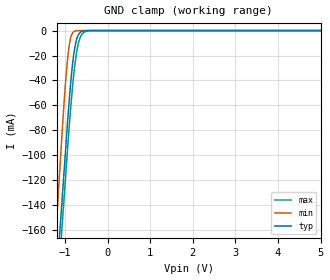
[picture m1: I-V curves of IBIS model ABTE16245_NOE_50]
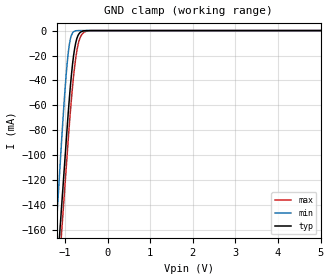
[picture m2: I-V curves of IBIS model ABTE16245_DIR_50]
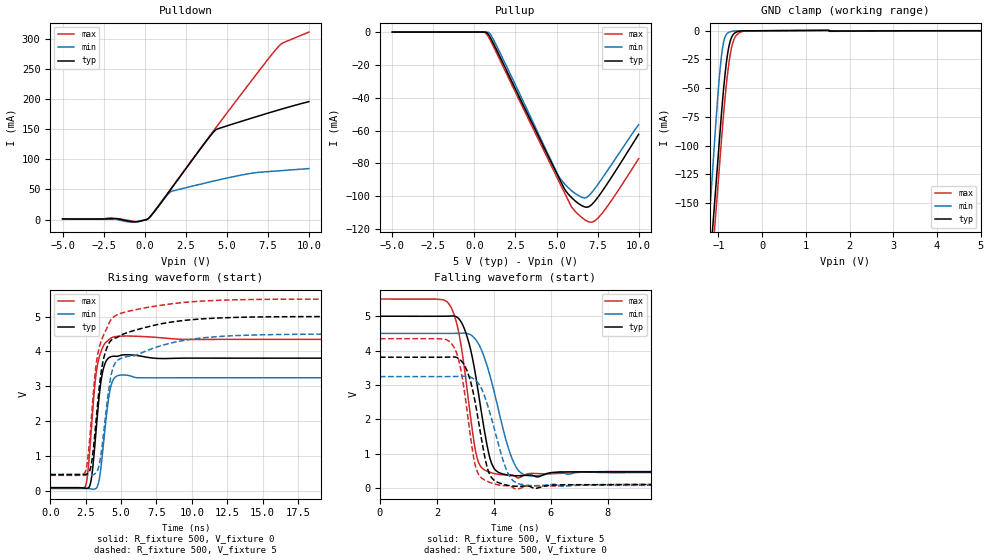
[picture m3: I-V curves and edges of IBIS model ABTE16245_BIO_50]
| TEXAS INSTRUMENTS INCORPORATED
| Standard Linear and Logic Group
| IBIS Model of SN74ABTE16245
| 16-BIT INCIDENT-WAVE SWITCHING BUS TRANSCEIVERS WITH 3-STATE OUTPUTS
| This file contains package information for the following:
|  TSSOP 48-pin (DGG) package as [Component] ABTE16245_DGG
|  SSOP 48-pin (DL) package as [Component] ABTE16245_DL
| This device can be powered at the following Vccs:
|  5 volt Vcc
| This file provides unique models under the [Model Selector] for each Vcc.
| For operation at a specific Vcc, select the appropriate model after each
| [Model Selector] keyword.
[IBIS Ver]   3.2
[Comment char]  |_char
[File Name]   sn74abte16245.ibs
[File Rev]   1.1 | a_die
[Date]   April 19, 2002
[Source]   Data created from TI-SPICE simulations at TI-SLL.
[Notes]   The following is an IBIS list for the ABTE16245.
   Please contact sllibis@ti.com with questions and
   comments concerning SLL IBIS models.
   -Non-monotonic data in ground-clamp due to bus-hold
   -C_comp values are taken at a different test condition than
   the data sheet.
   -Power clamp data deleted as there is no power-clamp diode.
   -Non-monotonic data in pullup data due to resistor at output.
[Disclaimer] Property of Texas Instruments Incorporated.  Unauthorized
   reproduction and/or distribution is strictly prohibited.
   This product is protected under copyright law.
   Created  2002, (C) Copyright  2002, Texas Instruments
   Incorporated, All Rights Reserved
   UNLESS THERE IS A SIGNED, WRITTEN AGREEMENT TO THE
   CONTRARY, TEXAS INSTRUMENTS (TI) IS PROVIDING THE IBIS
   MODELS  AND WITHOUT ANY WARRANTY, EXPRESSED OR
   IMPLIED.  TI assumes no liability for:
   1) the accuracy of the IBIS models provided to your
   company;
   2) the proper functioning of these IBIS Models in your
   design or for any resulting applications; or
   3) infringement of patents, copyrights or intellectual
   property rights resulting from your use of these IBIS
   models.
   TI provides IBIS Models as a service to our customers.
   You and your company shall not distribute, sell or give
   these models to anyone else without prior written
   permission from TI.
   TI reserves the right to make changes to our products or
   to discontinue any semiconductor product or service
   without notice, and advises our customers to obtain the
   latest version of relevant information to verify, before
   placing orders, that the information being relied on is
   current.
   Please be aware that your receipt and use of the IBIS
   information provided shall serve as acceptance of these
   terms and conditions.  If you do not accept these terms,
   you should return or destroy the IBIS models and any
   other accompanying information immediately.
| Component ABTE16245_DGG 48-pin TSSOP
[Component]   ABTE16245_DGG
[Manufacturer]   Texas Instruments, Inc.
[Package]
|   typ   min   max
R_pkg   4.400e-02   3.800e-02   5.100e-02
L_pkg   3.019e-09   2.486e-09   4.099e-09
C_pkg   5.070e-13   3.340e-13   8.090e-13
[Pin]   signal_name   model_name   R_pin   L_pin   C_pin
1   1DIR   ABTE16245_DIR   4.100e-02   4.017e-09   7.590e-13
2   1B1   ABTE16245_BIO   4.200e-02   3.737e-09   7.920e-13
3   2B1   ABTE16245_BIO   4.200e-02   3.480e-09   6.610e-13
4   GND   GND   3.800e-02   3.131e-09   5.750e-13
5   1B2   ABTE16245_BIO   4.700e-02   3.122e-09   5.660e-13
6   2B2   ABTE16245_BIO   4.300e-02   2.948e-09   5.040e-13
7   VCC   POWER   4.500e-02   2.845e-09   3.970e-13
8   1B3   ABTE16245_BIO   4.900e-02   2.835e-09   3.940e-13
9   2B3   ABTE16245_BIO   4.800e-02   2.715e-09   3.780e-13
10   GND   GND   5.000e-02   2.664e-09   3.630e-13
11   1B4   ABTE16245_BIO   5.000e-02   2.585e-09   3.480e-13
12   2B4   ABTE16245_BIO   4.900e-02   2.550e-09   3.370e-13
13   1B5   ABTE16245_BIO   4.900e-02   2.541e-09   3.360e-13
14   2B5   ABTE16245_BIO   5.000e-02   2.574e-09   3.480e-13
15   GND   GND   4.900e-02   2.618e-09   3.590e-13
16   1B6   ABTE16245_BIO   4.600e-02   2.671e-09   3.750e-13
17   2B6   ABTE16245_BIO   4.500e-02   2.754e-09   3.890e-13
18   VCC   POWER   4.400e-02   2.823e-09   4.500e-13
19   1B7   ABTE16245_BIO   4.200e-02   2.968e-09   5.030e-13
20   2B7   ABTE16245_BIO   5.100e-02   3.108e-09   5.350e-13
21   GND   GND   4.200e-02   3.175e-09   5.870e-13
22   1B8   ABTE16245_BIO   4.100e-02   3.449e-09   6.780e-13
23   2B8   ABTE16245_BIO   4.400e-02   3.766e-09   8.040e-13
24   2DIR   ABTE16245_DIR   4.300e-02   4.065e-09   7.610e-13
25   NOE   ABTE16245_NOE   4.100e-02   3.994e-09   7.570e-13
26   2A8   ABTE16245_AIO   3.900e-02   3.649e-09   7.890e-13
27   1A8   ABTE16245_AIO   3.800e-02   3.362e-09   6.600e-13
28   GND   GND   3.800e-02   3.082e-09   5.740e-13
29   2A7   ABTE16245_AIO   4.400e-02   2.990e-09   5.220e-13
30   1A7   ABTE16245_AIO   4.100e-02   2.917e-09   4.950e-13
31   VCC   POWER   4.300e-02   2.820e-09   4.480e-13
32   2A6   ABTE16245_AIO   4.300e-02   2.699e-09   3.850e-13
33   1A6   ABTE16245_AIO   4.500e-02   2.628e-09   3.720e-13
34   GND   GND   4.600e-02   2.556e-09   3.560e-13
35   2A5   ABTE16245_AIO   4.600e-02   2.495e-09   3.440e-13
36   1A5   ABTE16245_AIO   4.700e-02   2.487e-09   3.340e-13
37   2A4   ABTE16245_AIO   4.700e-02   2.490e-09   3.350e-13
38   1A4   ABTE16245_AIO   4.600e-02   2.486e-09   3.430e-13
39   GND   GND   4.500e-02   2.566e-09   3.560e-13
40   2A3   ABTE16245_AIO   4.400e-02   2.639e-09   3.740e-13
41   1A3   ABTE16245_AIO   4.300e-02   2.701e-09   3.860e-13
42   VCC   POWER   4.300e-02   2.817e-09   4.500e-13
43   2A2   ABTE16245_AIO   4.100e-02   2.935e-09   5.010e-13
44   1A2   ABTE16245_AIO   4.700e-02   3.035e-09   5.290e-13
45   GND   GND   4.300e-02   3.171e-09   5.890e-13
46   2A1   ABTE16245_AIO   4.000e-02   3.415e-09   6.820e-13
47   1A1   ABTE16245_AIO   4.300e-02   3.741e-09   8.090e-13
48   VCCBIAS   POWER   4.400e-02   4.099e-09   7.640e-13
| Component ABTE16245_DL 48-pin SSOP
[Component]   ABTE16245_DL
[Manufacturer]   Texas Instruments, Inc.
[Package]
|   typ   min   max
R_pkg   4.800e-02   3.800e-02   5.300e-02
L_pkg   6.046e-09   5.084e-09   7.968e-09
C_pkg   8.130e-13   5.690e-13   1.157e-12
[Pin]   signal_name   model_name   R_pin   L_pin   C_pin
1   1DIR   ABTE16245_DIR   4.600e-02   7.968e-09   1.017e-12
2   1B1   ABTE16245_BIO   4.400e-02   7.299e-09   1.157e-12
3   2B1   ABTE16245_BIO   4.300e-02   6.765e-09   1.058e-12
4   GND   GND   4.100e-02   6.269e-09   9.330e-13
5   1B2   ABTE16245_BIO   3.800e-02   5.856e-09   8.290e-13
6   2B2   ABTE16245_BIO   4.600e-02   5.802e-09   7.900e-13
7   VCC   POWER   5.000e-02   5.656e-09   7.380e-13
8   1B3   ABTE16245_BIO   5.300e-02   5.500e-09   6.430e-13
9   2B3   ABTE16245_BIO   5.200e-02   5.304e-09   6.060e-13
10   GND   GND   5.300e-02   5.189e-09   5.830e-13
11   1B4   ABTE16245_BIO   5.100e-02   5.084e-09   5.690e-13
12   2B4   ABTE16245_BIO   5.300e-02   5.862e-09   8.330e-13
13   1B5   ABTE16245_BIO   5.300e-02   5.862e-09   8.330e-13
14   2B5   ABTE16245_BIO   5.100e-02   5.084e-09   5.690e-13
15   GND   GND   5.300e-02   5.189e-09   5.830e-13
16   1B6   ABTE16245_BIO   5.200e-02   5.304e-09   6.060e-13
17   2B6   ABTE16245_BIO   5.300e-02   5.500e-09   6.430e-13
18   VCC   POWER   5.000e-02   5.656e-09   7.380e-13
19   1B7   ABTE16245_BIO   4.600e-02   5.802e-09   7.900e-13
20   2B7   ABTE16245_BIO   3.800e-02   5.856e-09   8.290e-13
21   GND   GND   4.100e-02   6.269e-09   9.330e-13
22   1B8   ABTE16245_BIO   4.300e-02   6.765e-09   1.058e-12
23   2B8   ABTE16245_BIO   4.400e-02   7.299e-09   1.157e-12
24   2DIR   ABTE16245_DIR   4.600e-02   7.968e-09   1.017e-12
25   NOE   ABTE16245_NOE   4.600e-02   7.968e-09   1.017e-12
26   2A8   ABTE16245_AIO   4.400e-02   7.299e-09   1.157e-12
27   1A8   ABTE16245_AIO   4.300e-02   6.765e-09   1.058e-12
28   GND   GND   4.100e-02   6.269e-09   9.330e-13
29   2A7   ABTE16245_AIO   3.800e-02   5.856e-09   8.290e-13
30   1A7   ABTE16245_AIO   4.600e-02   5.802e-09   7.900e-13
31   VCC   POWER   5.000e-02   5.656e-09   7.380e-13
32   2A6   ABTE16245_AIO   5.300e-02   5.500e-09   6.430e-13
33   1A6   ABTE16245_AIO   5.200e-02   5.304e-09   6.060e-13
34   GND   GND   5.300e-02   5.189e-09   5.830e-13
35   2A5   ABTE16245_AIO   5.100e-02   5.084e-09   5.690e-13
36   1A5   ABTE16245_AIO   5.300e-02   5.862e-09   8.330e-13
37   2A4   ABTE16245_AIO   5.300e-02   5.862e-09   8.330e-13
38   1A4   ABTE16245_AIO   5.100e-02   5.084e-09   5.690e-13
39   GND   GND   5.300e-02   5.189e-09   5.830e-13
40   2A3   ABTE16245_AIO   5.200e-02   5.304e-09   6.060e-13
41   1A3   ABTE16245_AIO   5.300e-02   5.500e-09   6.430e-13
42   VCC   POWER   5.000e-02   5.656e-09   7.380e-13
43   2A2   ABTE16245_AIO   4.600e-02   5.802e-09   7.900e-13
44   1A2   ABTE16245_AIO   3.800e-02   5.856e-09   8.290e-13
45   GND   GND   4.100e-02   6.269e-09   9.330e-13
46   2A1   ABTE16245_AIO   4.300e-02   6.765e-09   1.058e-12
47   1A1   ABTE16245_AIO   4.400e-02   7.299e-09   1.157e-12
48   VCCBIAS   POWER   4.600e-02   7.967e-09   1.017e-12
| Model ABTE16245_NOE
[Model Selector]   ABTE16245_NOE
ABTE16245_NOE_50   5 volt Vcc
| Model ABTE16245_DIR
[Model Selector]   ABTE16245_DIR
ABTE16245_DIR_50   5 volt Vcc
| Model ABTE16245_BIO
[Model Selector]   ABTE16245_BIO
ABTE16245_BIO_50   5 volt Vcc
| Model ABTE16245_AIO
[Model Selector]   ABTE16245_AIO
ABTE16245_AIO_50   5 volt Vcc
| Models and submodels in the file (4): ABTE16245_NOE_50 (Input), ABTE16245_DIR_50 (Input), ABTE16245_BIO_50 (I/O), ABTE16245_AIO_50 (I/O)
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[Model]   ABTE16245_NOE_50
Model_type  Input
Vinl=0.8
Vinh=2.0
| variable   typ   min   max
C_comp   3.08pF   2.43pF   4.35pF
[Temperature Range]   40   -40   100
| Ambient temperature   25   -40   85
[Voltage range]   5   4.5   5.5
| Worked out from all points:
|   GND clamp passes 1 mA (typ) near -0.62 V on its own axis
[GND Clamp]
| ABTE16245_NOE_50
|   Voltage   I(typ)   I(min)   I(max)
-5V       -2.047A    -2.272A    -2.046A
-1.225V   -210.9mA   -168.2mA   -231.3mA
-1.19V    -194mA     -148.7mA   -214.5mA
-1.13V    -164.9mA   -115.5mA   -185.7mA
-1.075V   -138.2mA   -85.02mA   -159.3mA
-1V       -101.9mA   -47.04mA   -123.3mA
-925mV    -65.91mA   -17.88mA   -87.3mA
-850mV    -35.54mA   -3.716mA   -54.84mA
-775mV    -14.51mA   -457.2uA   -29.06mA
-650mV    -1.663mA   -1.98uA    -5.988mA
-450mV    -7.8uA     -255.5pA   -199.2uA
5V        31.82pA    20.18pA    989.6pA
[Model]   ABTE16245_DIR_50
Model_type  Input
Vinl=1.4
Vinh=1.6
| variable   typ   min   max
C_comp   2.59pF   2.09pF   3.84pF
[Temperature Range]   40   -40   100
| Ambient temperature   25   -40   85
[Voltage range]   5   4.5   5.5
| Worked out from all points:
|   GND clamp passes 1 mA (typ) near -0.62 V on its own axis
[GND Clamp]
| ABTE16245_DIR_50
|   Voltage   I(typ)   I(min)   I(max)
-5V       -2.047A    -2.272A    -2.046A
-1.225V   -210.9mA   -168.2mA   -231.3mA
-1.19V    -194mA     -148.7mA   -214.5mA
-1.13V    -164.9mA   -115.5mA   -185.7mA
-1.075V   -138.2mA   -85.02mA   -159.3mA
-1V       -101.9mA   -47.04mA   -123.3mA
-925mV    -65.91mA   -17.88mA   -87.3mA
-850mV    -35.54mA   -3.716mA   -54.84mA
-775mV    -14.51mA   -457.2uA   -29.06mA
-650mV    -1.663mA   -1.98uA    -5.988mA
-450mV    -7.8uA     -255.5pA   -199.2uA
5V        31.82pA    20.18pA    989.6pA
[Model]   ABTE16245_BIO_50
Model_type  I/O
Vinl=1.4
Vinh=1.6
Enable   Active-Low
Vref =   0
Rref =   500
Cref =   50p
Vmeas =   1.5
| variable   typ   min   max
C_comp   6.03pF   4.66pF   8.45pF
| C_pullup   4.28pF   2.83pF   5.48pF
| C_pulldown   2.96pF   0.08pF   6.64pF
| C_tri-state   6.03pF   4.66pF   8.45pF
[Temperature Range]   40   -40   100
| Ambient temperature   25   -40   85
[Voltage range]   5   4.5   5.5
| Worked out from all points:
|   slope of the pulldown table from 0 to 0.75 V, typ, clamps not added: 37.7 ohm
|   slope of the pullup table from 0 to 0.75 V, typ, clamps not added: 2.29 kohm
|   GND clamp passes 1 mA (typ) near -0.58 V on its own axis
|   rising waveform, R_fixture 500, V_fixture 0: 20-80 % time 512ps typ, 516ps min, 540ps max; typ from 0.089 V to 3.81 V
|   falling waveform, R_fixture 500, V_fixture 5: 20-80 % time 567ps typ, 762ps min, 504ps max; typ from 5 V to 0.464 V
|   rising waveform, R_fixture 500, V_fixture 5: 20-80 % time 903ps typ, 981ps min, 1.01ns max; typ from 0.464 V to 5 V
|   falling waveform, R_fixture 500, V_fixture 0: 20-80 % time 505ps typ, 662ps min, 451ps max; typ from 3.81 V to 0.089 V
[GND Clamp]
| ABTE16245_BIO_50
|   Voltage   I(typ)   I(min)   I(max)
-5V       -2.171A    -2.386A    -2.177A
-1.25V    -230.4mA   -187.8mA   -252.5mA
-1.205V   -208mA     -162.3mA   -230.2mA
-1.12V    -165.8mA   -114.3mA   -188.3mA
-1.075V   -143.5mA   -88.9mA    -166.2mA
-1V       -106.4mA   -50.18mA   -129.3mA
-925mV    -69.61mA   -20.32mA   -92.4mA
-825mV    -29.91mA   -3.518mA   -49.23mA
-750mV    -11.96mA   -1.135mA   -25.53mA
-625mV    -1.954mA   -189.4uA   -6.015mA
-405mV    -89.46uA   -67.31uA   -275.3uA
5V        102.4pA    95.39pA    2.804nA
[Pulldown]
| ABTE16245_BIO_50
|   Voltage   I(typ)   I(min)   I(max)
-5V       1.029mA    1.295mA    822uA
-2.06V    1.405mA    2.828mA    912.9uA
-685mV    -3.652mA   -4.356mA   -2.879mA
170mV     687.5uA    636.9uA    995.1uA
530mV     11.26mA    10.94mA    11.97mA
1.585V    50.02mA    46.35mA    50.69mA
3.68V     127.9mA    60.71mA    128.7mA
4.335V    149.2mA    64.88mA    152.7mA
6.535V    168.8mA    77.13mA    232mA
8.19V     182.5mA    81.12mA    288.9mA
8.455V    184.6mA    81.66mA    294.2mA
10V       196.1mA    84.77mA    311.7mA
[Pullup]
| ABTE16245_BIO_50
|   Voltage   I(typ)   I(min)   I(max)
-5V       -7.069pA   -6.238pA   -6.06pA
695mV     -85.21uA   -164.5nA   -714.2uA
930mV     -2.641mA   -762.6uA   -4.304mA
1.27V     -9.131mA   -6.722mA   -11.03mA
5.14V     -88.55mA   -87.89mA   -90.74mA
5.53V     -96.18mA   -92.83mA   -98.68mA
5.935V    -100.9mA   -96.75mA   -106.7mA
6.65V     -106.2mA   -100.9mA   -113.8mA
7.135V    -105.1mA   -97.8mA    -115.7mA
7.59V     -99.63mA   -91.75mA   -112.6mA
8.44V     -87mA      -79.32mA   -101.2mA
10V       -62.26mA   -56.42mA   -77.11mA
[Ramp]
| ABTE16245_BIO_50
| variable   typ   min   max
dV/dt_r   2.30/5.38E-10   1.96/5.41E-10   2.61/5.71E-10
dV/dt_f   2.81/5.87E-10   2.50/7.89E-10   3.13/5.23E-10
R_load = 500
[Rising Waveform]
| ABTE16245_BIO_50
R_fixture =   500
C_fixture =   0
L_fixture =   0
V_fixture =   0
V_fixture_min = 0
V_fixture_max = 0
|   Time   V(typ)   V(min)   V(max)
0s        88.56mV    66.68mV    94.96mV
2.485ns   75.49mV    67.38mV    140.9mV
2.66ns    77.14mV    65.61mV    558.8mV
2.895ns   328.9mV    53.93mV    1.735V
3.135ns   1.244V     52.85mV    2.976V
3.325ns   2.149V     124.7mV    3.59V
3.74ns    3.483V     1.275V     4.145V
4.09ns    3.8V       2.564V     4.313V
4.37ns    3.856V     3.12V      4.399V
24.99ns   3.805V     3.242V     4.345V
[Falling Waveform]
| ABTE16245_BIO_50
R_fixture =   500
C_fixture =   0
L_fixture =   0
V_fixture =   5
V_fixture_min = 4.5
V_fixture_max = 5.5
|   Time   V(typ)   V(min)   V(max)
0s        5V         4.5V       5.5V
2.26ns    5V         4.498V     5.465V
2.8ns     4.894V     4.505V     4.371V
3.135ns   4.181V     4.478V     2.358V
3.405ns   3.027V     4.267V     886mV
3.78ns    1.151V     3.501V     479mV
4.03ns    538.1mV    2.724V     413mV
4.63ns    358.3mV    863.6mV    381.5mV
5.16ns    368.5mV    358.7mV    403.8mV
24.99ns   463.8mV    445.2mV    471.3mV
[Rising Waveform]
| ABTE16245_BIO_50
R_fixture =   500
C_fixture =   0
L_fixture =   0
V_fixture =   5
V_fixture_min = 4.5
V_fixture_max = 5.5
|   Time   V(typ)   V(min)   V(max)
0s        463.7mV    445.1mV    471.2mV
2.475ns   470.9mV    445.1mV    548.4mV
2.665ns   503.7mV    444.7mV    979.2mV
2.905ns   782.4mV    450.1mV    2.096V
3.36ns    2.558V     608.2mV    3.931V
3.86ns    3.935V     1.993V     4.552V
4.275ns   4.307V     3.27V      4.901V
4.67ns    4.392V     3.708V     5.039V
11.01ns   4.939V     4.397V     5.449V
24.99ns   5V         4.5V       5.5V
[Falling Waveform]
| ABTE16245_BIO_50
R_fixture =   500
C_fixture =   0
L_fixture =   0
V_fixture =   0
V_fixture_min = 0
V_fixture_max = 0
|   Time   V(typ)   V(min)   V(max)
0s        3.806V     3.242V     4.345V
2.5ns     3.813V     3.243V     4.212V
2.77ns    3.763V     3.248V     3.701V
3.03ns    3.458V     3.251V     2.413V
3.275ns   2.767V     3.183V     948.7mV
3.43ns    2.075V     3.066V     441.6mV
3.875ns   353.3mV    2.136V     152.8mV
4.4ns     89.26mV    610.8mV    63.04mV
4.765ns   47.53mV    158.3mV    -34.79mV
24.99ns   89mV       67.15mV    95.33mV
